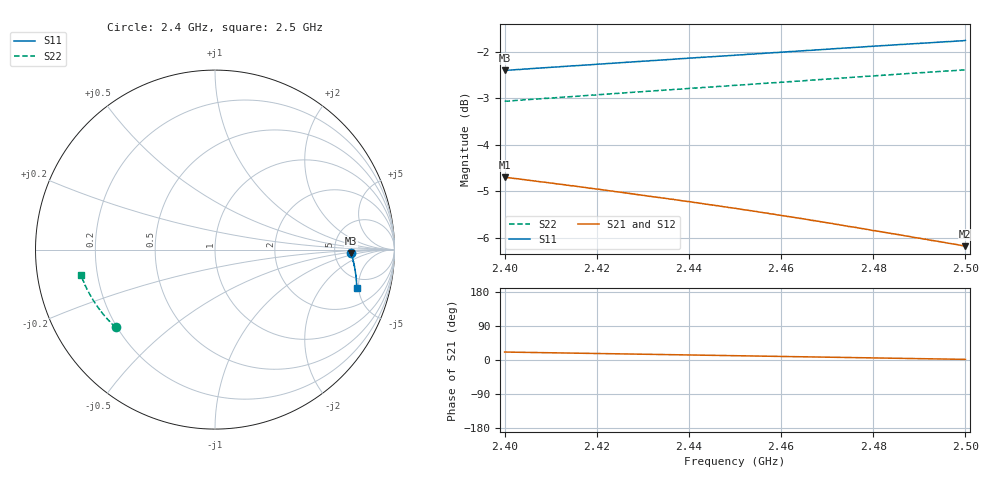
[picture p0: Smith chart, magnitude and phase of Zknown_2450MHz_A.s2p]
!Agilent Technologies,N5242A,MY49421279,A.09.90.21
!Agilent N5242A: A.09.90.21
!Date: Monday, January 30, 2023
!Caliblation kit: 85033D 3.5mm Calibration Kit
!DUT Connector Gender Port1: male
!DUT Connector Gender Port2: female
!S2P File: Measurements: S11, S21, S12, S22:
# Hz S  dB  R 50
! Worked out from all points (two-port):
!   1001 points, 2.4 GHz to 2.5 GHz, reference 50 ohm
!   highest |S21| = -4.70 dB at 2.4001 GHz (marker M1); lowest = -6.2 dB at 2.4999 GHz (marker M2)
!   |S21| within 3 dB of the highest: start of sweep to end of sweep
!   lowest |S11| = -2.4 dB at 2.4 GHz (marker M3), VSWR 7.29, Z = 361 - j35.6 ohm
!   |S11| at or under -10 dB: nowhere
!   |S22| runs from -3.1 to -2.4 dB; largest |S21 - S12| = 0.0026
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2.4e9  -2.40 -1.6  -4.70 21.0  -4.67 20.9  -3.06 -142.0
2.4001e9  -2.40 -1.6  -4.70 21.0  -4.67 20.9  -3.06 -142.0
2.4006e9  -2.40 -1.7  -4.71 20.9  -4.68 20.8  -3.06 -142.2
2.4061e9  -2.36 -2.4  -4.78 19.8  -4.75 19.8  -3.02 -143.7
2.4129e9  -2.31 -3.2  -4.86 18.5  -4.83 18.4  -2.97 -145.5
2.4167e9  -2.29 -3.7  -4.91 17.8  -4.88 17.7  -2.95 -146.6
2.4186e9  -2.28 -4.0  -4.93 17.4  -4.91 17.3  -2.94 -147.1
2.4243e9  -2.24 -4.7  -5.01 16.3  -4.98 16.2  -2.89 -148.6
2.4311e9  -2.20 -5.6  -5.11 15.0  -5.08 14.9  -2.85 -150.5
2.4334e9  -2.18 -5.9  -5.13 14.6  -5.11 14.5  -2.83 -151.2
2.4401e9  -2.13 -6.8  -5.23 13.3  -5.20 13.1  -2.79 -153.0
2.45e9  -2.07 -8.1  -5.37 11.4  -5.35 11.2  -2.72 -155.7
2.4568e9  -2.02 -9.0  -5.47 10.0  -5.45 9.9  -2.67 -157.6
2.4667e9  -1.96 -10.3  -5.63 8.1  -5.60 8.0  -2.60 -160.3
2.4724e9  -1.92 -11.1  -5.72 7.0  -5.69 6.9  -2.57 -161.8
2.4783e9  -1.89 -11.9  -5.82 5.9  -5.79 5.7  -2.52 -163.5
2.4834e9  -1.86 -12.6  -5.90 4.9  -5.88 4.7  -2.49 -164.9
2.4918e9  -1.81 -13.8  -6.04 3.3  -6.02 3.1  -2.44 -167.1
2.4959e9  -1.78 -14.4  -6.11 2.5  -6.10 2.3  -2.41 -168.3
2.4994e9  -1.76 -14.9  -6.17 1.8  -6.16 1.6  -2.39 -169.2
2.4999e9  -1.76 -15.0  -6.18 1.7  -6.17 1.5  -2.39 -169.4
2.5e9  -1.75 -15.0  -6.18 1.6  -6.17 1.5  -2.39 -169.4
